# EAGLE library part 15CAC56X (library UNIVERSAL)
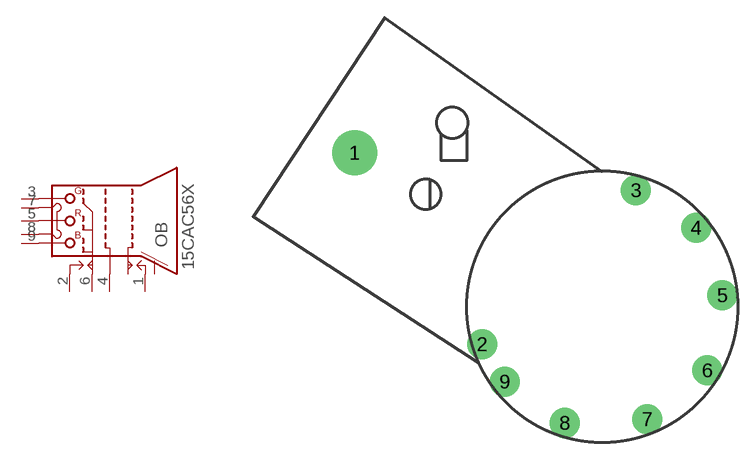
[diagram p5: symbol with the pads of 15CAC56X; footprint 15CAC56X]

Designator prefix OB

## 15CAC56X  [15CAC56X]
1  1
2  2
3  3
4  4
5  5
6  6
7  7
8  8
9  9

## Footprint 15CAC56X (pad centres in mm)
drill 0.813 pad 3.81: 1 -20.955,13.018
drill 0.813 pad 2.54: 2 -10.16,-3.175; 3 2.857,9.842; 4 7.938,6.668; 5 10.16,0.953; 6 8.89,-5.397; 7 3.81,-9.525; 8 -3.175,-9.842; 9 -8.255,-6.35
